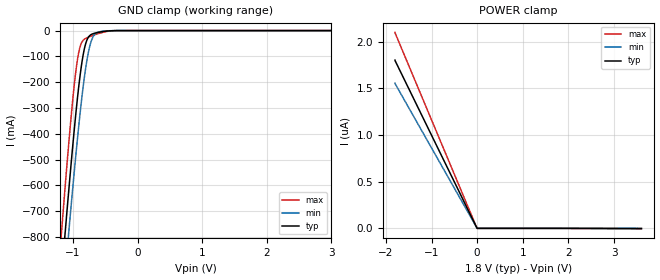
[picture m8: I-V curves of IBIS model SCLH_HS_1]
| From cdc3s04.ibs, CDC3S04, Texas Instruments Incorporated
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[Model]   SCLH_HS_1
Model_type   Input
Vinl = 540.000mV
Vinh = 1.260V
|   typ   min   max
C_comp   831.7fF   816.4fF   849.7fF
[Voltage Range]   1.800V   1.650V   1.950V
[Temperature Range]   32.0   85.0   -40.0
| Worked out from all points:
|   GND clamp passes 1 mA (typ) near -0.43 V on its own axis
[GND Clamp]
|   Voltage   I(typ)   I(min)   I(max)
-1.8V     -2.926A    -3.001A    -2.86A
-1.194V   -998.6mA   -1.149A    -829.1mA
-1.172V   -932.9mA   -1.086A    -760.4mA
-1.129V   -803mA     -960.3mA   -625.3mA
-1.089V   -683.5mA   -844.1mA   -502.1mA
-1.055V   -586.1mA   -748.7mA   -403.4mA
-975.2mV  -368.4mA   -531.3mA   -196.5mA
-917.1mV  -228.5mA   -383.1mA   -91.3mA
-822.6mV  -68.47mA   -177.3mA   -33.19mA
-720mV    -15.43mA   -42.07mA   -21.41mA
-451.4mV  -1.281mA   -681.2uA   -2.378mA
3.599V    0A         0A         0A
[POWER Clamp]
|   Voltage   I(typ)   I(min)   I(max)
-1.8V     1.802uA    1.555uA    2.099uA
-1.791V   1.788uA    1.543uA    2.084uA
0V        0A         0A         0A
3.599V    -2.683nA   -148.5pA   -3.293nA
